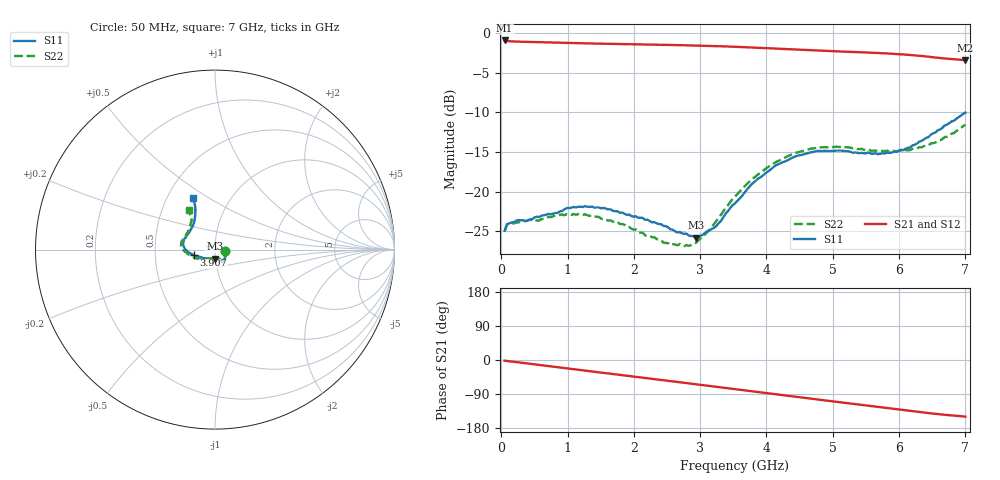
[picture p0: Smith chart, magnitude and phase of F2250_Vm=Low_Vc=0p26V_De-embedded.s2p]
! Integrated Device Technology
! Corporate Headquarters
! 6024 Silver Creek Valley Road
! San Jose, CA 95138  USA
! Phone:  1-408-284-8200
! Toll Free:  1-800-223-1366
! Webpage:  http://www.idt.com/
! Timing and RF Division
! 515 Groton Road, Suite 102
! Westford, MA 01886-6024
! Device:  F2250
! Description: Voltage Variable RF Attenuator
! Frequency:  50.0 -  6000.00 MHz
! Package:  3x3 mm Thin QFN Plastic Package: 16 pin
! Ports:  2 RF, 3 DC
!  Pin  1  = GND
!  Pin  2  = NC
!  Pin  3  = RF1  = Port 1
!  Pin  4  = NC
!  Pin  5  = GND
!  Pin  6  = GND
!  Pin  7  = GND
!  Pin  8  = GND
!  Pin  9  = NC
!  Pin 10  = RF2  = Port 2
!  Pin 11  = NC
!  Pin 12  = GND
!  Pin 13  = GND
!  Pin 14  = VCNTRL
!  Pin 15  = VDD
!  Pin 16  = VMODE
! Vcntrl:  0.260 Volts
! Vmode:  +0.000 Volts
! Vdd:  +3.30  Volts
! Current:  1.109 mA
! Data:  The device was measured on a the F2250 evaluation board which has
!  individual transmission lines to the RF pins.  Data was collected
!  using a calibrated network analyzer.  The evaluation board was
!  de-embedded using a TRL calibration technique.
!  The reference plane is the edge of the package pin.
! Misc:  SN 10
!  Action Tracker AT0258
! Date Measured:  2014-11-26
! Date:  2015-10-15  MJV
! Note:
!  Integrated Device Technology supplies this data as a sample of measured
!  data at the package pin for this product.  Your particular data for this
!  product may vary.
!  Data was taken at 25 degrees C.
!  Integrated Device Technology reserves the right to change this data at anytime.
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# GHz S dB R 50
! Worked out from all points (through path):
!   201 points, 50 MHz to 7 GHz, reference 50 ohm
!   highest |S21| = -0.94 dB at 50 MHz (marker M1); lowest = -3.4 dB at 7 GHz (marker M2)
!   group delay of S21, straight-line fit = 60 ps
!   lowest |S11| = -25.8 dB at 2.934 GHz (marker M3), VSWR 1.11, Z = 49.6 - j5.1 ohm
!   |S11| at or under -10 dB: start of sweep to end of sweep
!   |S22| runs from -26.9 to -11.6 dB; largest |S21 - S12| = 0.00032
!   S11 on the Smith chart (normalised r, x): 50 MHz: 1.12, -0.02; 3.907 GHz: 0.79, -0.05; 7 GHz: 0.67, +0.43
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0.05  -24.93 -9.5  -0.94 -1.8  -0.94 -1.8  -25.05 -10.0
0.08475  -24.12 -9.5  -1.01 -2.5  -1.01 -2.5  -24.18 -9.3
0.15425  -23.90 -11.7  -1.05 -4.0  -1.05 -4.0  -23.93 -11.0
0.57125  -23.19 -29.7  -1.15 -13.1  -1.15 -13.1  -23.66 -30.2
0.884  -22.48 -45.4  -1.22 -19.9  -1.22 -19.9  -22.91 -46.5
1.2315  -21.93 -55.5  -1.29 -27.4  -1.29 -27.4  -22.91 -59.4
1.75275  -22.49 -62.2  -1.39 -38.4  -1.38 -38.4  -23.79 -66.5
2.37825  -24.09 -63.0  -1.48 -51.8  -1.47 -51.8  -26.09 -68.1
2.552  -24.76 -67.2  -1.50 -55.6  -1.50 -55.6  -26.75 -73.6
2.83  -25.55 -82.4  -1.55 -61.7  -1.55 -61.7  -26.85 -92.7
2.93425  -25.81 -91.4  -1.58 -64.0  -1.57 -64.0  -26.49 -101.5
3.21225  -24.56 -120.9  -1.64 -70.2  -1.64 -70.2  -24.04 -127.3
3.525  -21.48 -147.5  -1.73 -77.1  -1.73 -77.1  -20.64 -146.2
3.76825  -19.12 -160.7  -1.82 -82.5  -1.82 -82.5  -18.51 -156.5
3.90725  -18.20 -165.1  -1.88 -85.5  -1.88 -85.5  -17.62 -162.7
4.1505  -16.64 -173.3  -1.98 -90.8  -1.98 -90.8  -16.23 -171.3
4.7065  -14.99 172.5  -2.19 -102.8  -2.19 -102.8  -14.57 175.7
5.15825  -14.85 161.8  -2.35 -112.6  -2.35 -112.6  -14.33 166.6
5.85325  -15.12 138.6  -2.60 -127.5  -2.60 -127.5  -14.95 151.5
6.166  -14.43 127.7  -2.77 -134.3  -2.77 -134.3  -14.77 142.6
6.444  -13.12 119.4  -2.98 -140.1  -2.98 -140.1  -14.15 133.3
7  -10.04 113.1  -3.42 -149.4  -3.42 -149.4  -11.58 123.8
